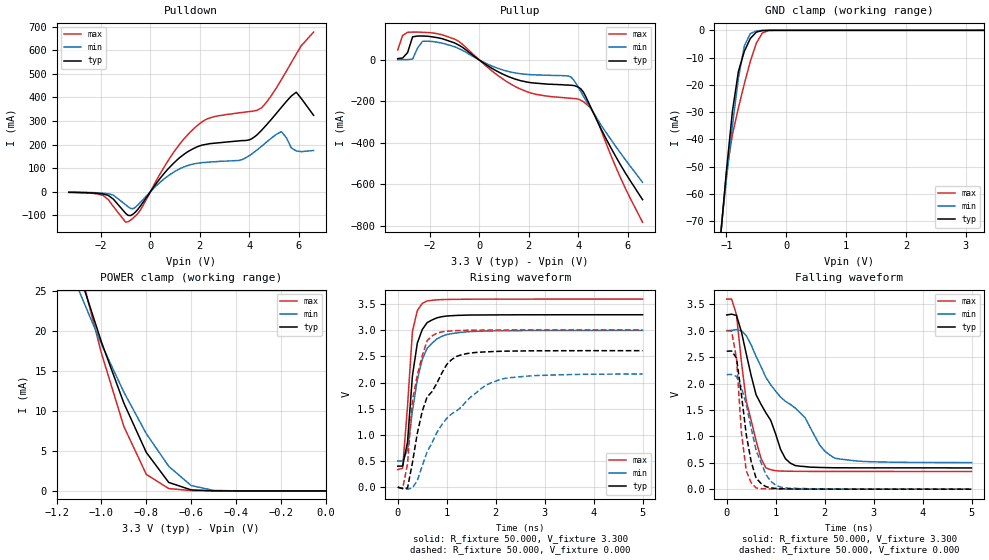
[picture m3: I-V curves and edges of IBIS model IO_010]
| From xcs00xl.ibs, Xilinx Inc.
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|   Model IO_010
[Model]   IO_010
Model_type   I/O
Polarity   Non-Inverting
Enable   Active-Low
Vinl =   0.800V
Vinh =   2.000V
Vmeas =   1.650V
Cref =  50.000pF
Rref =   1.000M
Vref =  0.000V
C_comp   5.300pF   3.500pF   6.800pF
[Temperature Range]   50.000   100.000   0.000
[Voltage Range]   3.300V   3.000V   3.600V
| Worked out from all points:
|   slope of the pulldown table from 0 to 0.495 V, typ, clamps not added: 7.07 ohm
|   slope of the pullup table from 0 to 0.495 V, typ, clamps not added: 12.6 ohm
|   GND clamp passes 1 mA (typ) near -0.52 V on its own axis
|   POWER clamp passes 1 mA (typ) near -0.69 V on its own axis
|   rising waveform, R_fixture 50.000, V_fixture 3.300: 20-80 % time 185ps typ, 288ps min, 145ps max; typ from 0.402 V to 3.3 V
|   rising waveform, R_fixture 50.000, V_fixture 0.000: 20-80 % time 542ps typ, 991ps min, 258ps max; typ from 0 V to 2.61 V
|   falling waveform, R_fixture 50.000, V_fixture 3.300: 20-80 % time 659ps typ, 1.19ns min, 341ps max; typ from 3.3 V to 0.403 V
|   falling waveform, R_fixture 50.000, V_fixture 0.000: 20-80 % time 242ps typ, 372ps min, 160ps max; typ from 2.61 V to 0.001 V
[Pulldown]
| voltage   I(typ)   I(min)   I(max)
-3.3V     -2.3mA     -1.8mA     -2.8mA
-1.9V     -9.7mA     -6.1mA     -16.3mA
-900mV    -100mA     -63.86mA   -127mA
-400mV    -59.92mA   -44.53mA   -76.62mA
700mV     94.99mA    66.07mA    129mA
1.6V      175mA      114mA      252mA
2.3V      202mA      125mA      309mA
3.6V      216mA      133mA      335mA
4.5V      261mA      193mA      356mA
5.3V      358mA      255mA      476mA
5.9V      422mA      173mA      584mA
6.6V      324mA      175mA      677mA
[Pullup]
| voltage   I(typ)   I(min)   I(max)
-3.3V     6.59mA     1.22mA     48.5mA
-3.1V     9.75mA     1.52mA     119mA
-2.7V     112mA      4.46mA     135mA
-2.3V     116mA      90.3mA     134mA
-1.7V     108mA      86.06mA    127mA
-800mV    69.91mA    53.59mA    87.42mA
1.6V      -97.48mA   -65.22mA   -137mA
3.6V      -121mA     -77.38mA   -184mA
4.2V      -154mA     -173mA     -201mA
4.7V      -278mA     -272mA     -271mA
5.7V      -505mA     -448mA     -567mA
6.6V      -675mA     -591mA     -784mA
[GND_clamp]
| voltage   I(typ)   I(min)   I(max)
-3.3V     -539mA     -461mA     -635mA
-1.1V     -76.29mA   -74.81mA   -76.3mA
-1V       -51.66mA   -54.6mA    -52.25mA
-900mV    -29.77mA   -35.09mA   -38.23mA
-800mV    -15.1mA    -17.65mA   -28.49mA
-700mV    -7.645mA   -5.66mA    -19.53mA
-600mV    -2.968mA   -1.205mA   -11.34mA
-500mV    -649uA     -202uA     -4.68mA
-400mV    -83.34uA   -28.89uA   -976uA
-300mV    -8.303uA   -3.567uA   -95.2uA
3.3V      90.2nA     487nA      4.544uA
[POWER_clamp]
| voltage   I(typ)   I(min)   I(max)
-3.3V     51.86mA    10.89mA    181mA
-3.1V     70.08mA    13.61mA    230mA
-3V       85.17mA    15.89mA    249mA
-2.9V     108mA      19.33mA    255mA
-2.8V     138mA      24.96mA    249mA
-1.1V     27.32mA    25.08mA    28.22mA
-1V       18.65mA    18.39mA    17.25mA
-900mV    11mA       12.37mA    8.069mA
-800mV    4.821mA    7.171mA    2.071mA
-700mV    1.064mA    3.083mA    296uA
-600mV    127uA      671uA      39.67uA
0V        90.2nA     23.33nA    5.636uA
[Ramp]
| variable   typ   min   max
dV/dt_r   1.567/0.517n   1.299/0.991n   1.805/0.280n
dV/dt_f   1.738/0.629n   1.497/1.169n   1.958/0.348n
R_load = 50.000
[Rising Waveform]
R_fixture = 50.000
V_fixture = 3.300
V_fixture_min = 3.000
V_fixture_max = 3.600
L_fixture = 0.000H
C_fixture = 0.000F
| time   V(typ)   V(min)   V(max)
0s        402mV      503mV      335mV
100ps     404mV      499mV      362mV
200ps     861mV      715mV      1.55V
300ps     2.127V     1.456V     2.977V
400ps     2.755V     2.052V     3.377V
500ps     3.013V     2.442V     3.515V
600ps     3.147V     2.656V     3.563V
800ps     3.239V     2.837V     3.584V
1.2ns     3.285V     2.95V      3.593V
5ns       3.298V     2.998V     3.598V
[Rising Waveform]
R_fixture = 50.000
V_fixture = 0.000
V_fixture_min = 0.000
V_fixture_max = 0.000
L_fixture = 0.000H
C_fixture = 0.000F
| time   V(typ)   V(min)   V(max)
0s        0V         0V         0V
100ps     -26.7mV    -19.53mV   -26.7mV
200ps     -16.57mV   -38.29mV   440mV
300ps     466mV      -13.62mV   1.653V
400ps     1.032V     124mV      2.145V
600ps     1.726V     675mV      2.8V
700ps     1.827V     849mV      2.892V
1.2ns     2.5V       1.459V     2.995V
2.1ns     2.599V     2.062V     3.006V
5ns       2.611V     2.165V     3.008V
[Falling Waveform]
R_fixture = 50.000
V_fixture = 3.300
V_fixture_min = 3.000
V_fixture_max = 3.600
L_fixture = 0.000H
C_fixture = 0.000F
| time   V(typ)   V(min)   V(max)
0s        3.3V       3V         3.6V
100ps     3.315V     3.008V     3.601V
200ps     3.291V     3.023V     3.307V
400ps     2.562V     2.907V     1.668V
600ps     1.79V      2.516V     918mV
800ps     1.448V     2.117V     404mV
1.1ns     755mV      1.745V     344mV
1.3ns     493mV      1.606V     340mV
2.2ns     406mV      590mV      337mV
5ns       403mV      504mV      336mV
[Falling Waveform]
R_fixture = 50.000
V_fixture = 0.000
V_fixture_min = 0.000
V_fixture_max = 0.000
L_fixture = 0.000H
C_fixture = 0.000F
| time   V(typ)   V(min)   V(max)
0s        2.613V     2.169V     3.009V
100ps     2.618V     2.173V     2.991V
200ps     2.486V     2.135V     2.482V
300ps     1.799V     1.931V     1.079V
400ps     1.032V     1.606V     350mV
500ps     522mV      1.157V     121mV
600ps     211mV      738mV      23.43mV
800ps     48.67mV    280mV      7.014mV
1.1ns     8.649mV    40.88mV    3.193mV
5ns       737uV      819uV      657uV
